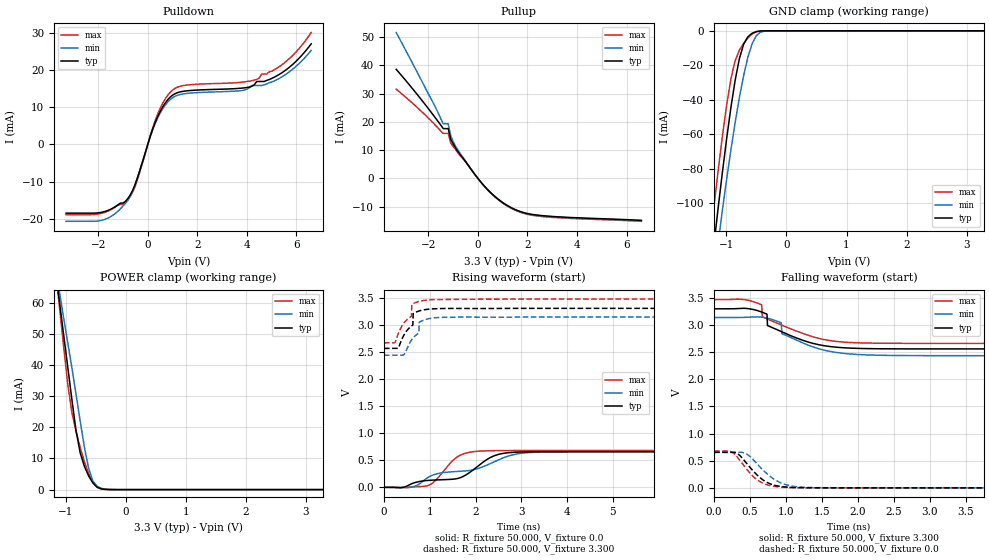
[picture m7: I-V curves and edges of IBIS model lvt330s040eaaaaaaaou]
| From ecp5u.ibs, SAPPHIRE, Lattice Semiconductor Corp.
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|   Model lvt330s040eaaaaaaaou
[Model] lvt330s040eaaaaaaaou
Model_type  Output
Polarity   Non-Inverting
Enable   Active-Low
Vmeas =  1.650V
Cref =  0.0F
Rref =  1.000M
Vref =  0.0V
C_comp   5.000pF   4.000pF   5.500pF
[Temperature Range]   25.000   0.125k   -40.000
[Voltage Range]   3.300V   3.140V   3.470V
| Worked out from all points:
|   slope of the pulldown table from 0 to 0.495 V, typ, clamps not added: 56.4 ohm
|   slope of the pullup table from 0 to 0.495 V, typ, clamps not added: 101 ohm
|   GND clamp passes 1 mA (typ) near -0.54 V on its own axis
|   POWER clamp passes 1 mA (typ) near -0.49 V on its own axis
|   rising waveform, R_fixture 50.000, V_fixture 0.0: 20-80 % time 1.24ns typ, 1.67ns min, 436ps max; typ from 0 V to 0.656 V
|   rising waveform, R_fixture 50.000, V_fixture 3.300: 20-80 % time 255ps typ, 254ps min, 297ps max; typ from 2.56 V to 3.3 V
|   falling waveform, R_fixture 50.000, V_fixture 3.300: 20-80 % time 521ps typ, 488ps min, 617ps max; typ from 3.3 V to 2.56 V
|   falling waveform, R_fixture 50.000, V_fixture 0.0: 20-80 % time 289ps typ, 327ps min, 275ps max; typ from 0.656 V to 0 V
[Pulldown]
|Voltage   I(typ)   I(min)   I(max)
-3.3V     -18.5mA    -20.69mA   -18.92mA
-1.8V     -18.18mA   -20.31mA   -18.41mA
-800mV    -14.52mA   -15.03mA   -14.85mA
-500mV    -10.57mA   -10.59mA   -11.09mA
300mV     5.903mA    5.609mA    6.426mA
600mV     10.05mA    9.542mA    11.01mA
1V        13.21mA    12.54mA    14.59mA
1.6V      14.4mA     13.7mA     15.95mA
4V        15.26mA    14.8mA     16.87mA
4.4V      16.89mA    15.82mA    17.46mA
5.5V      19.62mA    18.48mA    21.81mA
6.6V      27.02mA    25.25mA    30.04mA
[Pullup]
|Voltage   I(typ)   I(min)   I(max)
-3.3V     38.64mA    51.66mA    31.61mA
-2.3V     28.07mA    35.04mA    23.89mA
-1.4V     17.64mA    19.38mA    15.96mA
-1.2V     17.64mA    19.38mA    15.96mA
-1.1V     13.94mA    15.18mA    12.64mA
-1V       12.25mA    12.98mA    11.27mA
-800mV    9.415mA    9.937mA    8.988mA
100mV     -1.098mA   -1.08mA    -1.128mA
900mV     -7.923mA   -7.9mA     -8.094mA
1.6V      -11.37mA   -11.43mA   -11.61mA
2.3V      -12.88mA   -12.99mA   -13.19mA
6.6V      -14.84mA   -14.99mA   -15.18mA
[GND_clamp]
|Voltage   I(typ)   I(min)   I(max)
-3.3V     -912.7mA   -861.5mA   -922.5mA
-1.27V    -145.6mA   -163.6mA   -123.5mA
-1.2V     -123.4mA   -142.6mA   -101.4mA
-1.13V    -102mA     -122.4mA   -80.37mA
-1.06V    -81.56mA   -103.5mA   -60.64mA
-920mV    -44.4mA    -68.93mA   -27.87mA
-780mV    -16.18mA   -38.86mA   -11.24mA
-710mV    -7.839mA   -26.12mA   -7.318mA
-570mV    -1.464mA   -7.654mA   -1.852mA
-430mV    -105.8uA   -801.1uA   -99.73uA
-290mV    -1.56uA    -33.42uA   -868.4nA
3.28V     0A         0A         0A
[POWER_clamp]
|Voltage   I(typ)   I(min)   I(max)
-3.28V    471.5mA    421.2mA    516.6mA
-1.18V    71.72mA    72.75mA    72.14mA
-1.11V    60.88mA    63.98mA    59.38mA
-970mV    39.73mA    47.46mA    34.21mA
-900mV    29.12mA    39.28mA    24.89mA
-830mV    19.01mA    30.67mA    18.7mA
-760mV    11.8mA     22.01mA    13.51mA
-620mV    4.416mA    6.921mA    5.219mA
-550mV    2.174mA    2.865mA    2.414mA
-480mV    813uA      1.102mA    758.3uA
-200mV    3.62uA     22.61uA    424nA
3.3V      0A         0A         0A
[Ramp]
| variable   typ   min   max
dV/dt_r   0.396/1.202n   0.395/1.651n   0.409/0.445n
dV/dt_f   0.442/0.612n   0.421/0.595n   0.490/0.683n
R_load = 50.000
[Rising Waveform]
R_fixture= 50.000
V_fixture= 0.0
V_fixture_min= 0.0
V_fixture_max= 0.0
|time   V(typ)   V(min)   V(max)
0s        0V         0V         0V
367ps     -7.331mV   -428.5uV   -6.523mV
605ps     65.93mV    6.006mV    4.646mV
977ps     128.2mV    189.2mV    37.86mV
1.131ns   135.5mV    244mV      131.3mV
1.584ns   158.3mV    291.1mV    550.2mV
2.031ns   375.6mV    340.6mV    664.4mV
2.488ns   603.9mV    501.4mV    676.8mV
3.238ns   654.6mV    644.2mV    678.1mV
10ns      655.9mV    653.9mV    678.1mV
[Rising Waveform]
R_fixture= 50.000
V_fixture= 3.300
V_fixture_min= 3.140
V_fixture_max= 3.470
|time   V(typ)   V(min)   V(max)
0s        2.561V     2.437V     2.663V
239ps     2.561V     2.437V     2.669V
436ps     2.807V     2.446V     3.028V
601ps     2.975V     2.713V     3.154V
607ps     2.978V     2.72V      3.373V
631ps     2.992V     2.747V     3.384V
637ps     3.2V       2.753V     3.387V
768ps     3.252V     3.042V     3.428V
950ps     3.282V     3.104V     3.454V
10ns      3.3V       3.14V      3.47V
[Falling Waveform]
R_fixture= 50.000
V_fixture= 3.300
V_fixture_min= 3.140
V_fixture_max= 3.470
|time   V(typ)   V(min)   V(max)
0s        3.3V       3.14V      3.47V
576ps     3.278V     3.153V     3.419V
662ps     3.241V     3.147V     3.373V
735ps     3.202V     3.13V      3.116V
742ps     2.993V     3.128V     3.112V
766ps     2.979V     3.12V      3.099V
933ps     2.881V     3.042V     3.003V
943ps     2.875V     2.842V     2.997V
1.853ns   2.578V     2.472V     2.682V
10ns      2.561V     2.437V     2.663V
[Falling Waveform]
R_fixture= 50.000
V_fixture= 0.0
V_fixture_min= 0.0
V_fixture_max= 0.0
|time   V(typ)   V(min)   V(max)
0s        655.9mV    653.9mV    678.1mV
250ps     657.3mV    653.8mV    659.2mV
340ps     616.5mV    656.1mV    538mV
433ps     482.4mV    635mV      376.9mV
566ps     279.2mV    488.7mV    182.9mV
695ps     131.6mV    307.8mV    76.88mV
842ps     47.3mV     152.5mV    25.5mV
982ps     16.75mV    64.59mV    8.601mV
1.599ns   547.9uV    1.446mV    569.3uV
10ns      0V         0V         0V
